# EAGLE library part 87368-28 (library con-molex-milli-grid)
RECEPTACAL
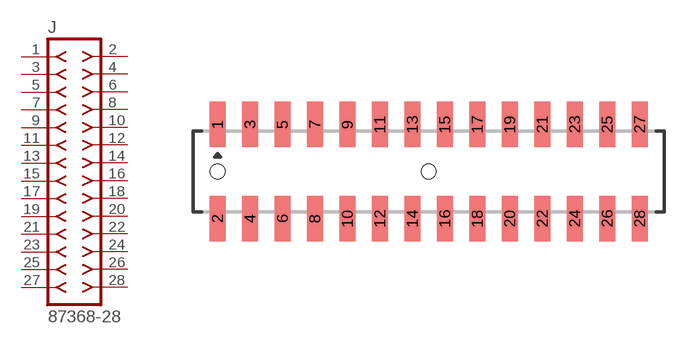
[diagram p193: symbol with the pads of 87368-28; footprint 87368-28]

Designator prefix J

## 87368-28  [87368-28]
1  1  pas
2  2  pas
3  3  pas
4  4  pas
5  5  pas
6  6  pas
7  7  pas
8  8  pas
9  9  pas
10  10  pas
11  11  pas
12  12  pas
13  13  pas
14  14  pas
15  15  pas
16  16  pas
17  17  pas
18  18  pas
19  19  pas
20  20  pas
21  21  pas
22  22  pas
23  23  pas
24  24  pas
25  25  pas
26  26  pas
27  27  pas
28  28  pas

## Footprint 87368-28 (pad centres in mm)
RECEPTACAL SMD Dual Row, Side Entry
smd 1 x 2.8: 1 -13,2.9; 2 -13,-2.9; 3 -11,2.9; 4 -11,-2.9; 5 -9,2.9; 6 -9,-2.9; 7 -7,2.9; 8 -7,-2.9; 9 -5,2.9; 10 -5,-2.9; 11 -3,2.9; 12 -3,-2.9; 13 -1,2.9; 14 -1,-2.9; 15 1,2.9; 16 1,-2.9; 17 3,2.9; 18 3,-2.9; 19 5,2.9; 20 5,-2.9; 21 7,2.9; 22 7,-2.9; 23 9,2.9; 24 9,-2.9; 25 11,2.9; 26 11,-2.9; 27 13,2.9; 28 13,-2.9
hole 0.914 at -13,0
hole 0.914 at 0,0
